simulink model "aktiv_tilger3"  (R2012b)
settings: Solver=ode45  StartTime=0.0  StopTime=10.0  RelTol=1e-3
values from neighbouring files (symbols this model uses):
  a11 = a11{:}    [aktiv_tilger_2.m]    (also in aktiv_tilger_3.m; aktiv_tilger_31.m)
  a12 = a12{:}    [aktiv_tilger_2.m]    (also in aktiv_tilger_3.m; aktiv_tilger_31.m)
  a21 = a21{:}    [aktiv_tilger_2.m]    (also in aktiv_tilger_3.m; aktiv_tilger_31.m)
  a22 = a22{:}    [aktiv_tilger_2.m]    (also in aktiv_tilger_3.m; aktiv_tilger_31.m)
  b11 = b11{:}    [aktiv_tilger_2.m]    (also in aktiv_tilger_3.m; aktiv_tilger_31.m)
  b12 = b12{:}    [aktiv_tilger_2.m]    (also in aktiv_tilger_3.m; aktiv_tilger_31.m)
  b21 = b21{:}    [aktiv_tilger_2.m]    (also in aktiv_tilger_3.m; aktiv_tilger_31.m)
  b22 = b22{:}    [aktiv_tilger_2.m]    (also in aktiv_tilger_3.m; aktiv_tilger_31.m)
  D = 0    [aktiv_tilger_1.m]    (also in aktiv_tilger_12.m; aktiv_tilger_3.m = 2000; aktiv_tilger_31.m; beobachter_1.m)
  fsig = 0.01    [aktiv_tilger_1.m]    (also in aktiv_tilger_12.m = 0.1; aktiv_tilger_2.m = 2; aktiv_tilger_3.m = 0.1; diff_filter_1.m = 1)
  I = 2000    [aktiv_tilger_1.m]    (also in aktiv_tilger_12.m; aktiv_tilger_3.m = 0; aktiv_tilger_31.m = 0; fuellstnd_2.m = 0.0225)
  P = 0    [aktiv_tilger_1.m]    (also in aktiv_tilger_12.m; aktiv_tilger_3.m; aktiv_tilger_31.m; fuellstnd_2.m = 0.09)
libraries: simulink x1

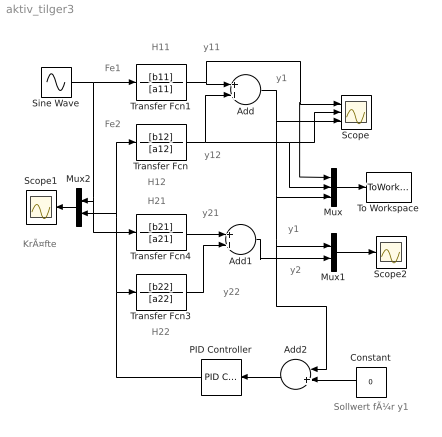
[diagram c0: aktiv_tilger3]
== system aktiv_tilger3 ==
  note: H22
  note: H21
  note: H12
  note: H11
  note: KrÃ¤fte
  note: y22
  note: y21
  note: y1
  note: Sollwert fÃ¼r y1
  note: y2
  note: Fe2
  note: Fe1
  note: y1
  note: y12
  note: y11
  Add : Sum
  Add1 : Sum
  Add2 : Sum  Inputs=-+
  Constant : Constant  Value=0
  Mux : Mux  Inputs=3
  Mux1 : Mux  Inputs=2
  Mux2 : Mux  Inputs=2
  PID Controller : simulink/Continuous/PID Controller  Controller=PID  TimeDomain=Continuous-time  SampleTime=1  IntegratorMethod=Forward Euler  FilterMethod=Forward Euler  Form=Parallel  P=P  I=I  D=D  N=100  InitialConditionSource=internal  InitialConditionForIntegrator=0  InitialConditionForFilter=0  ExternalReset=none  LimitOutput=off  UpperSaturationLimit=inf  LowerSaturationLimit=-inf  LinearizeAsGain=on  AntiWindupMode=none  Kb=1  TrackingMode=off  Kt=1  PParamMin=[]  PParamMax=[]  IParamMin=[]  IParamMax=[]  DParamMin=[]  DParamMax=[]  NParamMin=[]  NParamMax=[]  KbParamMin=[]  KbParamMax=[]  KtParamMin=[]  KtParamMax=[]  POutMin=[]  POutMax=[]  IOutMin=[]  IOutMax=[]  DOutMin=[]  DOutMax=[]  NOutMin=[]  NOutMax=[]  KbOutMin=[]  KbOutMax=[]  KtOutMin=[]  KtOutMax=[]  IntegratorOutMin=[]  IntegratorOutMax=[]  FilterOutMin=[]  FilterOutMax=[]  SumOutMin=[]  SumOutMax=[]  SumI1OutMin=[]  SumI1OutMax=[]  SumI2OutMin=[]  SumI2OutMax=[]  SumI3OutMin=[]  SumI3OutMax=[]  SumDOutMin=[]  SumDOutMax=[]  SaturationOutMin=[]  SaturationOutMax=[]  IntegratorContinuousStateAttributes=''  IntegratorStateMustResolveToSignalObject=off  IntegratorRTWStateStorageClass=Auto  FilterContinuousStateAttributes=''  FilterStateMustResolveToSignalObject=off  FilterRTWStateStorageClass=Auto
  Scope : Scope  NumInputPorts=3
  Scope1 : Scope
  Scope2 : Scope
  Sine Wave : Sin  Amplitude=0.5  Frequency=fsig*2*pi  SampleTime=0
  To Workspace : ToWorkspace  VariableName=y  SampleTime=-1  SaveFormat=Structure With Time
  Transfer Fcn : TransferFcn  Numerator=[b12]  Denominator=[a12]
  Transfer Fcn1 : TransferFcn  Numerator=[b11]  Denominator=[a11]
  Transfer Fcn3 : TransferFcn  Numerator=[b22]  Denominator=[a22]
  Transfer Fcn4 : TransferFcn  Numerator=[b21]  Denominator=[a21]
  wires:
  Sine Wave/1 -> Mux2/1, Transfer Fcn4/1, Transfer Fcn1/1
  Mux/1 -> To Workspace/1
  Transfer Fcn/1 -> Scope/2, Mux/2, Add/2
  Transfer Fcn1/1 -> Mux/1, Scope/1, Add/1
  Transfer Fcn4/1 -> Add1/1
  Transfer Fcn3/1 -> Add1/2
  Add1/1 -> Mux1/2
  Mux1/1 -> Scope2/1
  Add2/1 -> PID Controller/1
  Add/1 -> Mux/3, Add2/1, Mux1/1, Scope/3
  Constant/1 -> Add2/2
  Mux2/1 -> Scope1/1
  PID Controller/1 -> Mux2/2, Transfer Fcn/1, Transfer Fcn3/1
